FUNCTION FC 38 : VOID
TITLE =
VERSION : 0.1

BEGIN
NETWORK
TITLE =START TRASFERIMENTO PARAMETRI ACP600
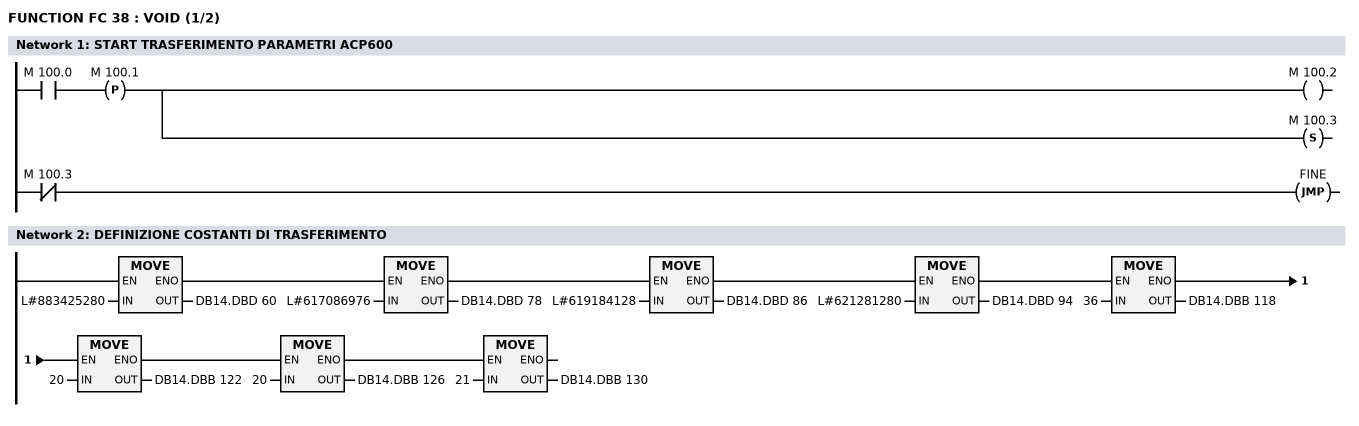
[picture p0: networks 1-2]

      U     M    100.0;
      FP    M    100.1;
      =     M    100.2;
      S     M    100.3;

      UN    M    100.3;
      SPB   FINE;


NETWORK
TITLE =DEFINIZIONE COSTANTI DI TRASFERIMENTO

      L     L#883425280;
      T     DB14.DBD   60;
      L     L#617086976;
      T     DB14.DBD   78;
      L     L#619184128;
      T     DB14.DBD   86;
      L     L#621281280;
      T     DB14.DBD   94;
      L     36;
      T     DB14.DBB  118;
      L     20;
      T     DB14.DBB  122;
      L     20;
      T     DB14.DBB  126;
      L     21;
      T     DB14.DBB  130;

NETWORK
TITLE =GESTIONE STEPS TRASFERIMENTO PARAMETRI ACP600
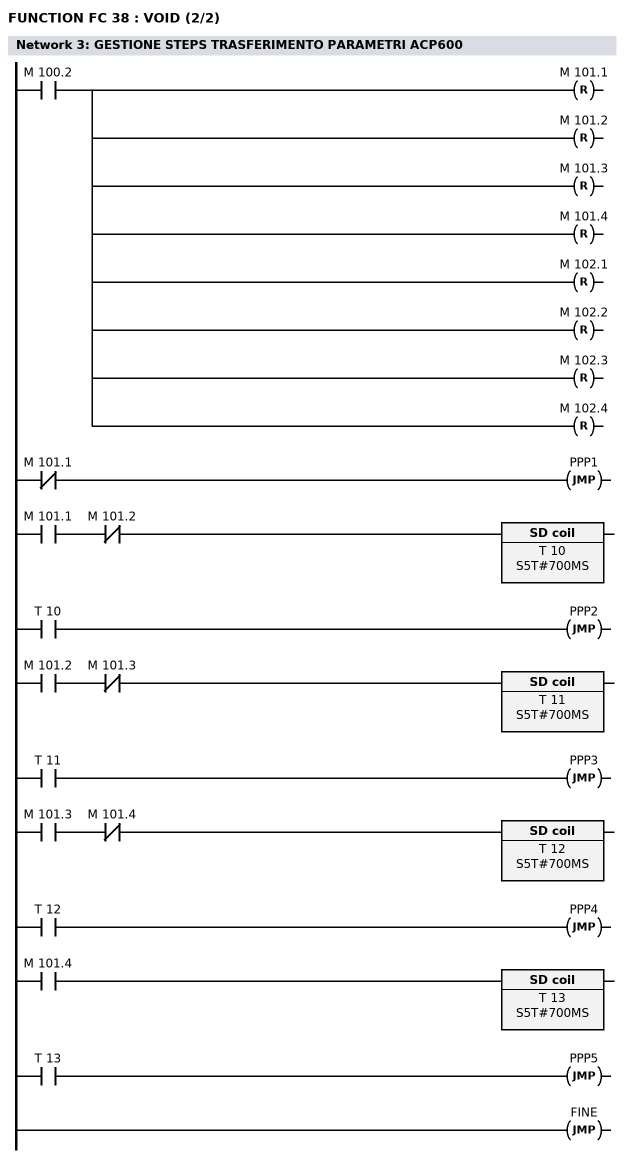
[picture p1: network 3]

      U     M    100.2;
      R     M    101.1;
      R     M    101.2;
      R     M    101.3;
      R     M    101.4;
      R     M    102.1;
      R     M    102.2;
      R     M    102.3;
      R     M    102.4;

      UN    M    101.1;
      SPB   PPP1;

      U     M    101.1;
      UN    M    101.2;
      L     S5T#700MS;
      SE    T     10;
      U     T     10;
      SPB   PPP2;

      U     M    101.2;
      UN    M    101.3;
      L     S5T#700MS;
      SE    T     11;
      U     T     11;
      SPB   PPP3;

      U     M    101.3;
      UN    M    101.4;
      L     S5T#700MS;
      SE    T     12;
      U     T     12;
      SPB   PPP4;

      U     M    101.4;
      L     S5T#700MS;
      SE    T     13;
      U     T     13;
      SPB   PPP5;
      SPA   FINE;

NETWORK
TITLE =PARAMETRO POSIZIONE

PPP1: L     DB14.DBD  134;
      L     L#52887;
      *D    ;
      L     1000;
      /D    ;
      T     DB14.DBD   64;

      CALL "DPWR_DAT" (
           LADDR                    := W#16#100,
           RECORD                   := P#DB14.DBX60.0 BYTE 8,
           RET_VAL                  := DB14.DBW   68);

      CALL "DPRD_DAT" (
           LADDR                    := W#16#100,
           RET_VAL                  := DB14.DBW   68,
           RECORD                   := P#DB14.DBX70.0 BYTE 8);

      S     M    101.1;
      SPA   FINE;

NETWORK
TITLE =PARAMETRO VELOCITA

PPP2: L     DB14.DBD   70;
      T     DB14.DBD  114;

      L     DB14.DBD  138;
      L     21835;
      *D    ;
      L     10000;
      /D    ;
      T     DB14.DBD   82;

      CALL "DPWR_DAT" (
           LADDR                    := W#16#100,
           RECORD                   := P#DB14.DBX78.0 BYTE 8,
           RET_VAL                  := DB14.DBW   68);

      CALL "DPRD_DAT" (
           LADDR                    := W#16#100,
           RET_VAL                  := DB14.DBW   68,
           RECORD                   := P#DB14.DBX70.0 BYTE 8);

      S     M    101.2;
      SPA   FINE;

NETWORK
TITLE =PARAMETRO ACCELERAZIONE

PPP3: L     DB14.DBD   70;
      T     DB14.DBD  102;

      CALL "DPWR_DAT" (
           LADDR                    := W#16#100,
           RECORD                   := P#DB14.DBX86.0 BYTE 8,
           RET_VAL                  := DB14.DBW   68);

      CALL "DPRD_DAT" (
           LADDR                    := W#16#100,
           RET_VAL                  := DB14.DBW   68,
           RECORD                   := P#DB14.DBX70.0 BYTE 8);

      S     M    101.3;
      SPA   FINE;

NETWORK
TITLE =PARAMETRO DECELERAZIONE

PPP4: L     DB14.DBD   70;
      T     DB14.DBD  106;

      L     DB14.DBD  142;
      L     -1;
      *D    ;
      T     DB14.DBD   98;
//
      CALL "DPWR_DAT" (
           LADDR                    := W#16#100,
           RECORD                   := P#DB14.DBX94.0 BYTE 8,
           RET_VAL                  := DB14.DBW   68);

      CALL "DPRD_DAT" (
           LADDR                    := W#16#100,
           RET_VAL                  := DB14.DBW   68,
           RECORD                   := P#DB14.DBX70.0 BYTE 8);

      S     M    101.4;
      SPA   FINE;

PPP5: L     DB14.DBD   70;
      T     DB14.DBD  110;

      CALL "DPRD_DAT" (
           LADDR                    := W#16#100,
           RET_VAL                  := DB14.DBW   68,
           RECORD                   := P#DB14.DBX70.0 BYTE 8);

      L     DB14.DBD   70;
      T     DB14.DBD  114;

NETWORK
TITLE =VERIFICA COMUNICAZIONE OK
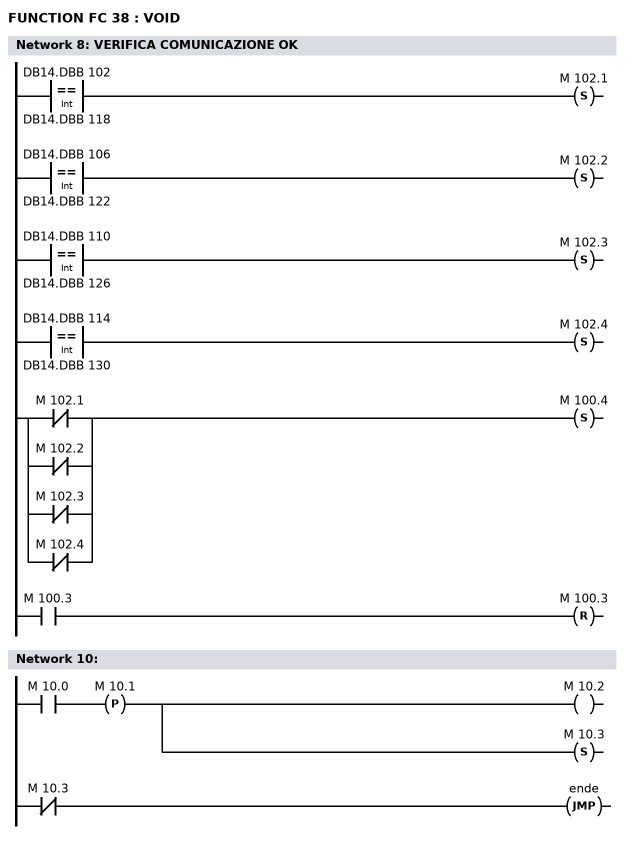
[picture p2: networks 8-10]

      L     DB14.DBB  102;
      L     DB14.DBB  118;
      ==I   ;
      S     M    102.1;

      L     DB14.DBB  106;
      L     DB14.DBB  122;
      ==I   ;
      S     M    102.2;

      L     DB14.DBB  110;
      L     DB14.DBB  126;
      ==I   ;
      S     M    102.3;

      L     DB14.DBB  114;
      L     DB14.DBB  130;
      ==I   ;
      S     M    102.4;

      U(    ;
      ON    M    102.1;
      ON    M    102.2;
      ON    M    102.3;
      ON    M    102.4;
      )     ;
      S     M    100.4;

      U     M    100.3;
      R     M    100.3;

NETWORK
TITLE =FINE TRASMISSIONE

FINE: NOP   0;

NETWORK
TITLE =

      U     M     10.0;
      FP    M     10.1;
      =     M     10.2;
      S     M     10.3;

      UN    M     10.3;
      SPB   ende;


NETWORK
TITLE =

//      U     A     42.7
//      =     M     10.0

      U     M     10.2;
      R     M     10.4;
      R     M     10.5;

      UN    M     10.4;
      SPB   m002;
      U     M     10.4;
      UN    M     10.5;
      L     S5T#700MS;
      SE    T      8;
      U     M     10.5;
      SPB   m006;
      U     T      8;
      SPB   m003;
      SPA   ende;
m002: NOP   0;
      L     W#16#203; //CW DATO 0000_0010_0000_0110
      T     DB14.DBW  158;

      CALL "DPWR_DAT" (
           LADDR                    := W#16#111,//= 273
           RECORD                   := P#DB14.DBX158.0 BYTE 2,
           RET_VAL                  := DB14.DBW   68);

//      CALL  "DPRD_DAT"
//       LADDR  :=W#16#130
//       RET_VAL:="DATI ENCODER".STAT17
//       RECORD :="DATI ENCODER".STAT42
      S     M     10.4;
      SPA   ende;
m003: NOP   0;

      L     W#16#200; //CW DATO 0000_0010_0000_0110
      T     DB14.DBW  158;

      CALL "DPWR_DAT" (
           LADDR                    := W#16#111,//= 273
           RECORD                   := P#DB14.DBX158.0 BYTE 2,
           RET_VAL                  := DB14.DBW   68);

//      CALL  "DPRD_DAT"
//       LADDR  :=W#16#130
//       RET_VAL:="DATI ENCODER".STAT17
//       RECORD :="DATI ENCODER".STAT42
      S     M     10.5;
      SPA   ende;
m006: U     M     10.3;
      R     M     10.3;


NETWORK
TITLE =

ende: NOP   0;

      CALL "DPRD_DAT" (
           LADDR                    := W#16#130,
           RET_VAL                  := DB14.DBW   68,
           RECORD                   := "ABBILD_AUSGÄNGE1");

END_FUNCTION

